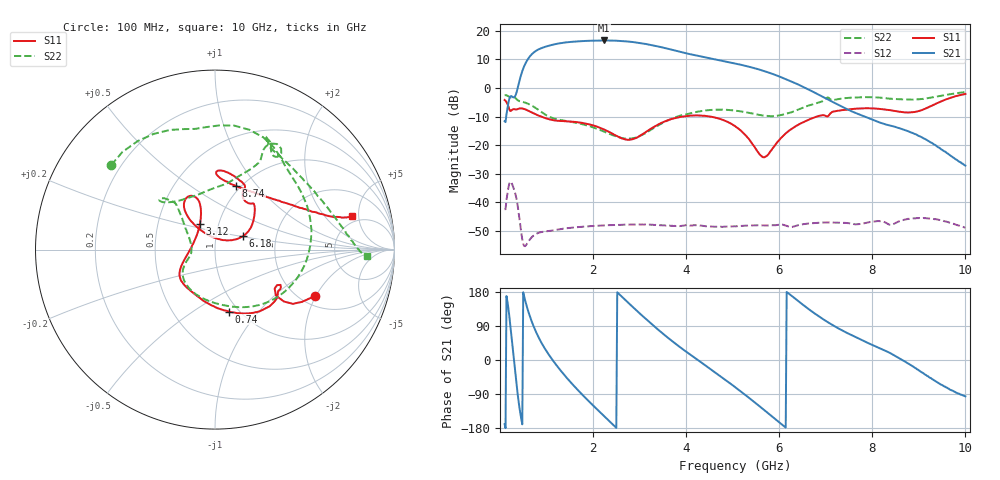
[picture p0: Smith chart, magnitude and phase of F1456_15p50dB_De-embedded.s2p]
! Integrated Device Technology
! Corporate Headquarters
! 6024 Silver Creek Valley Road
! San Jose, CA 95138  USA
! Phone:  1-408-284-8200
! Toll Free:  1-800-223-1366
! Webpage:  http://www.idt.com/
! Timing and RF Division
! 515 Groton Road, Suite 102
! Westford, MA 01886-6024
! Device:  F1456
! Description: 6-bit 0.5 dB Transmit Variable Gain Amplifier
! Frequency:  2100.0 -  2950.00 MHz
! Package:  6x6 mm Thin QFN Plastic Package: 28 pin
! State:  31
! Atten State:  15.5 dB
! Voltage:  +5.00 Volts
! Current:  216.991 mA
! Data:  The device was measured on a the F1455 evaluation board which has
!  individual transmission lines to the RF pins.  Data was collected
!  using a calibrated network analyzer.  The evaluation board was
!  de-embedded using a TRL calibration technique.
!  The reference plane is the edge of the package pin.
!  Pin  1 = CSb
!  Pin  2 = DATA
!  Pin  3 = CLK
!  Pin  4 = RSET
!  Pin  5 = GND
!  Pin  6 = RFIN  = Port 1
!  Pin  7 = GND
!  Pin  8 = NC
!  Pin  9 = NC
!  Pin 10 = NC
!  Pin 11 = NC
!  Pin 12 = NC
!  Pin 13 = NC
!  Pin 14 = /STBY
!  Pin 15 = GND
!  Pin 16 = RFOUT  = Port 2
!  Pin 17 = GND
!  Pin 18 = NC
!  Pin 19 = NC
!  Pin 20 = NC
!  Pin 21 = GND
!  Pin 22 = NC
!  Pin 23 = GND
!  Pin 24 = NC
!  Pin 25 = NC
!  Pin 26 = NC
!  Pin 27 = GND
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# GHz S dB R 50
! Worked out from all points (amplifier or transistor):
!   496 points, 100 MHz to 10 GHz, reference 50 ohm
!   highest |S21| = 16.6 dB at 2.24 GHz (marker M1)
!   |S21| within 3 dB of that: 843.9 MHz to 3.634 GHz (2.79 GHz wide, 125 % of centre)
!   unconditionally stable (mu >= 1): start of sweep to end of sweep
!   at 1.74 GHz: K = 18.06, MAG = 16.8 dB, |S12| = -48.5 dB
!   at 5.06 GHz: K = 39.24, MAG = 9.5 dB, |S12| = -48.3 dB
!   at 10 GHz: K = 340.83, MAG = -17.5 dB, |S12| = -48.8 dB
!   S11 on the Smith chart (normalised r, x): 100 MHz: 2.35, -1.98; 740 MHz: 0.90, -0.71; 3.12 GHz: 0.81, +0.24; 6.18 GHz: 1.35, +0.21; 8.74 GHz: 0.95, +0.78; 10 GHz: 4.22, +4.10
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0.1  -4.22 -25.1  -11.62 -169.1  -42.31 47.9  -2.55 140.8
0.32  -7.46 -32.0  -3.04 -20.1  -36.35 -147.7  -3.34 66.8
0.44  -7.13 -41.5  3.78 -142.7  -48.33 137.1  -4.70 38.3
0.58  -7.73 -59.2  9.52 139.8  -54.45 162.3  -5.36 6.9
0.74  -9.01 -77.2  12.57 83.9  -51.35 136.2  -6.70 -27.7
0.96  -10.48 -99.0  14.30 31.1  -50.14 95.3  -9.18 -67.4
1.18  -11.35 -116.2  15.26 -8.3  -49.65 70.1  -10.74 -95.4
1.48  -11.71 -132.8  16.01 -53.4  -48.88 45.0  -11.72 -123.1
1.76  -12.18 -143.5  16.34 -90.3  -48.46 26.8  -12.62 -139.7
2.24  -14.54 -159.4  16.58 -148.5  -47.99 0.7  -15.27 -157.4
2.64  -17.73 171.3  16.36 164.6  -47.80 -19.3  -17.55 -173.7
3.12  -15.58 120.2  15.38 110.0  -47.68 -43.1  -15.86 154.5
3.4  -12.78 109.9  14.47 79.9  -47.90 -56.6  -13.11 140.6
3.74  -10.64 108.8  13.15 46.0  -48.20 -70.8  -10.41 132.2
4.08  -9.69 113.7  11.80 15.1  -48.05 -86.2  -8.90 131.5
5.06  -13.44 130.0  8.51 -72.3  -48.33 -130.3  -7.93 138.3
5.64  -24.09 83.2  6.08 -128.4  -48.01 -162.9  -9.61 122.3
6.18  -15.32 25.7  2.76 177.7  -48.30 163.2  -8.86 83.8
6.7  -10.65 41.6  -1.12 128.2  -47.24 138.9  -5.79 64.7
8.36  -7.73 87.8  -13.03 19.9  -47.72 68.2  -3.73 62.4
8.74  -8.55 71.7  -14.95 -7.2  -45.86 61.5  -4.06 49.1
10  -2.10 13.7  -27.12 -96.0  -48.78 -24.0  -1.46 -2.6
